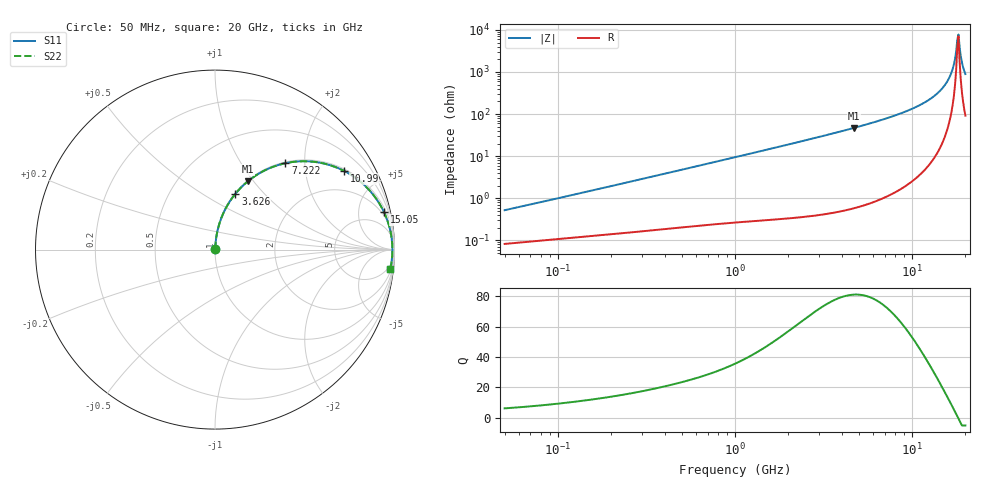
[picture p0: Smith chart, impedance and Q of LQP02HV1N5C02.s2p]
!Murata Part Number: LQP02HV1N5C02
!These Parameters are Measured in Series Mode Connection
!  o--[Z]--o
!Port1  Port2
!  o-------o
!Freq. Start=50[MHz] Stop=20[GHz], 401[Steps]
# Hz S RI R 50
!Freq.(Hz) S11(Real) S11(Imag) S21(Real) S21(Imag) S12(Real) S12(Imag) S22(Real) S22(Imag)
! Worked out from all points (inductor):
!   401 points, 50 MHz to 20 GHz, reference 50 ohm
!   read as one part in series: L = 1.62 nH near 51.52 MHz
!   highest Q = 81.1 at 4.678 GHz (marker M1), where L = 1.59 nH
!   self-resonance near 18.01 GHz
!   S11 on the Smith chart (normalised r, x): 50 MHz: 1.00, +0.01; 3.626 GHz: 1.01, +0.71; 7.222 GHz: 1.02, +1.60; 10.99 GHz: 1.07, +3.22; 15.05 GHz: 1.48, +8.85; 20 GHz: 3, -18
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5e7  0.00085 0.00514  0.9992 -0.00514  0.9992 -0.00514  0.00085 0.00514
1.364002e8  0.00138 0.0134  0.9986 -0.0134  0.9986 -0.0134  0.00138 0.0134
3.721004e8  0.00305 0.0355  0.9969 -0.0355  0.9969 -0.0355  0.00305 0.0355
1e9  0.0114 0.0931  0.9886 -0.0931  0.9886 -0.0931  0.0114 0.0931
2.728004e9  0.0668 0.2424  0.9332 -0.2424  0.9332 -0.2424  0.0668 0.2424
3.626126e9  0.1137 0.3111  0.8863 -0.3111  0.8863 -0.3111  0.1137 0.3111
4.677679e9  0.1824 0.3801  0.8176 -0.3801  0.8176 -0.3801  0.1824 0.3801
7.222371e9  0.3917 0.4813  0.6083 -0.4813  0.6083 -0.4813  0.3917 0.4813
7.442007e9  0.4114 0.4851  0.5886 -0.4851  0.5886 -0.4851  0.4114 0.4851
9.178299e9  0.5677 0.487  0.4323 -0.487  0.4323 -0.487  0.5677 0.487
1.098561e10  0.718 0.4392  0.282 -0.4392  0.282 -0.4392  0.718 0.4392
1.314879e10  0.8602 0.3309  0.1398 -0.3309  0.1398 -0.3309  0.8602 0.3309
1.504638e10  0.9413 0.2096  0.0587 -0.2096  0.0587 -0.2096  0.9413 0.2096
1.597544e10  0.9658 0.1469  0.0342 -0.1469  0.0342 -0.1469  0.9658 0.1469
1.670968e10  0.9786 0.0973  0.0214 -0.0973  0.0214 -0.0973  0.9786 0.0973
1.721783e10  0.9842 0.0635  0.0158 -0.0635  0.0158 -0.0635  0.9842 0.0635
1.774144e10  0.9875 0.0293  0.0125 -0.0293  0.0125 -0.0293  0.9875 0.0293
1.800918e10  0.9883 0.012  0.0117 -0.012  0.0117 -0.012  0.9883 0.012
1.828096e10  0.9884 -0.00519  0.0116 0.00519  0.0116 0.00519  0.9884 -0.00519
1.855685e10  0.988 -0.0224  0.012 0.0224  0.012 0.0224  0.988 -0.0224
1.940974e10  0.983 -0.0738  0.017 0.0738  0.017 0.0738  0.983 -0.0738
2e10  0.9768 -0.1075  0.0232 0.1075  0.0232 0.1075  0.9768 -0.1075
